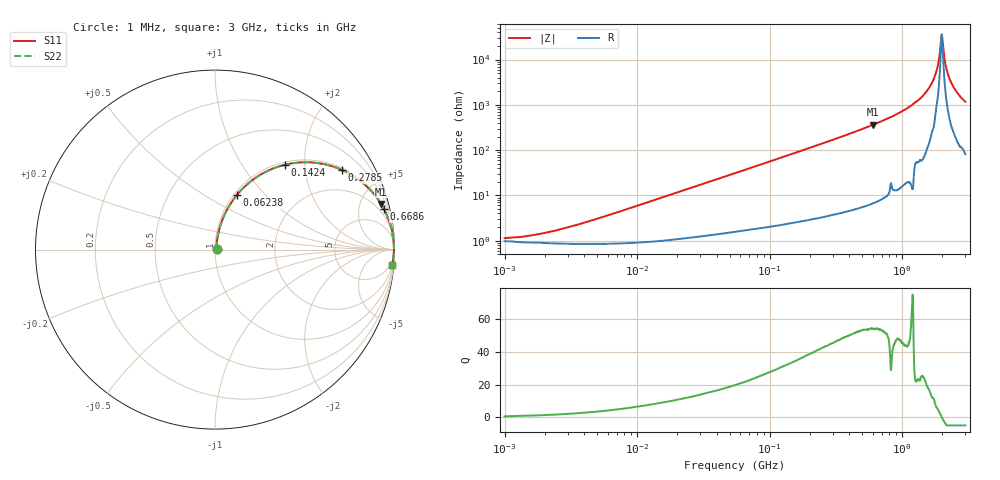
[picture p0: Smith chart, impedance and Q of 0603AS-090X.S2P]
!s-Parameter Generated by FASTRON Sdn. Bhd.
!FASTRON P/N : 0603AS-090X
!Keysight Technologies: E4991B_MY54100416_A.01.15
!Date created: Wed Oct 04 13:01:18 2023
!Version  : Rev01 Wed Oct 04 13:01:18 2023
!Data & Calibration Information:
!Freq	S11	S21	S12	S22
!PortZ  Port1:50+j0  Port2:50+j0
!When reading reference impedance value at option line is always used.
! Remarks : This data is being provided solely for informational purposes.
# Hz S dB R 50
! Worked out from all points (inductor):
!   1601 points, 1 MHz to 3 GHz, reference 50 ohm
!   read as one part in series: L = 93.7 nH near 4.354 MHz
!   highest Q = 54.2 at 601.9 MHz (marker M1), where L = 95.8 nH
!   self-resonance near 1.98 GHz
!   S11 on the Smith chart (normalised r, x): 1 MHz: 1.02, +0.01; 62.38 MHz: 1.03, +0.70; 142.4 MHz: 1.05, +1.59; 278.5 MHz: 1.07, +3.14; 668.6 MHz: 1.15, +8.24; 3 GHz: 3, -23
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1000000  -38.93 31.0  -0.08 -0.3  -0.08 -0.3  -38.93 31.0
3804036  -32.47 67.9  -0.08 -1.3  -0.08 -1.3  -32.47 67.9
1.447069e7  -21.57 78.6  -0.11 -4.8  -0.11 -4.8  -21.57 78.6
5.477226e7  -10.69 70.1  -0.52 -17.0  -0.52 -17.0  -10.69 70.1
6.238265e7  -9.69 68.2  -0.63 -19.1  -0.63 -19.1  -9.69 68.2
1.424433e8  -4.23 50.4  -2.26 -37.9  -2.26 -37.9  -4.23 50.4
2.083556e8  -2.50 40.0  -3.84 -48.6  -3.84 -48.6  -2.50 40.0
2.785165e8  -1.57 32.1  -5.48 -56.6  -5.48 -56.6  -1.57 32.1
6.018993e8  -0.36 15.3  -11.55 -73.6  -11.55 -73.6  -0.36 15.3
6.685918e8  -0.29 13.6  -12.58 -75.4  -12.58 -75.4  -0.29 13.6
7.925923e8  -0.19 10.9  -14.44 -77.9  -14.44 -77.9  -0.19 10.9
1.147801e9  -0.07 6.2  -19.39 -82.7  -19.39 -82.7  -0.07 6.2
1.542004e9  -0.03 2.8  -26.26 -84.2  -26.26 -84.2  -0.03 2.8
1.773925e9  -0.03 1.2  -33.20 -81.7  -33.20 -81.7  -0.03 1.2
1.855641e9  -0.02 0.8  -37.16 -78.1  -37.16 -78.1  -0.02 0.8
1.941122e9  -0.02 0.3  -45.20 -61.4  -45.20 -61.4  -0.02 0.3
1.990301e9  -0.02 -0.0  -51.10 1.0  -51.10 1.0  -0.02 -0.0
2.040726e9  -0.03 -0.3  -44.91 58.4  -44.91 58.4  -0.03 -0.3
2.177892e9  -0.03 -1.0  -35.04 78.5  -35.04 78.5  -0.03 -1.0
2.312676e9  -0.03 -1.7  -30.59 81.4  -30.59 81.4  -0.03 -1.7
2.607784e9  -0.05 -3.1  -25.35 82.1  -25.35 82.1  -0.05 -3.1
3e9  -0.08 -4.8  -21.44 81.1  -21.44 81.1  -0.08 -4.8
